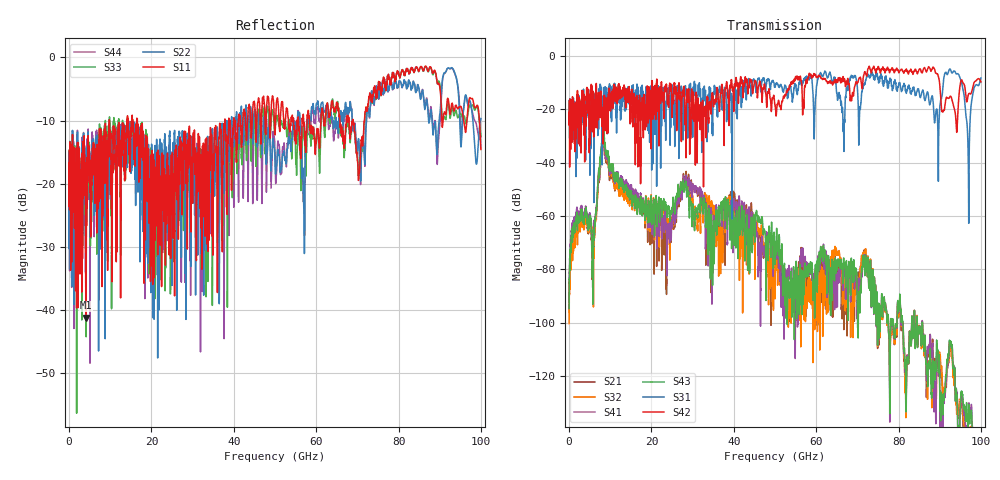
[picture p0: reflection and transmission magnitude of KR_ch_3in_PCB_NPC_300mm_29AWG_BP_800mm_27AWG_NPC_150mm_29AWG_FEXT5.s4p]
# GHz S RI R 45
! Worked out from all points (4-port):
!   4000 points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, 25 MHz to 100 GHz, reference 45 ohm
!   strongest paths, dB at 25 MHz, 25.02 GHz, 50.02 GHz, 75.03 GHz, 100 GHz:
!     S42: -21.2, -20.7, -18.6, -4.1, -9.8
!     S31: -21.3, -12.1, -11.5, -8.0, -8.3
!     S43: -94.7, -58.5, -72.8, -94.6, -158.5
!     S41: -92.2, -62.3, -71.0, -94.8, -150.9
!     S32: -100.3, -63.0, -83.5, -95.3, -162.7
!     S21: -96.2, -60.9, -74.2, -95.6, -162.4
!   lowest |S11| = -41.3 dB at 4.075 GHz (marker M1), VSWR 1.02, Z = 44.6 - j0.641 ohm
!   |S11| at or under -10 dB: start of sweep to 9.799 GHz; 9.805 GHz to 14.12 GHz (4.315 GHz wide, 36.1 % of centre); 16.58 GHz to 37.83 GHz (21.26 GHz wide, 78.1 % of centre)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
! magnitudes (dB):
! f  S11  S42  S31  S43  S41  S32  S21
! 25 MHz  -16.7  -21.2  -21.3  -94.7  -92.2  -100.3  -96.2
! 4.075 GHz  -41.3  -21.9  -35.0  -57.4  -56.6  -59.3  -59.0
! 8.375 GHz  -12.8  -19.1  -17.5  -28.2  -29.8  -29.5  -31.2
! 23.27 GHz  -24.1  -11.9  -24.6  -56.2  -59.1  -61.7  -61.0
! 28.6 GHz  -15.4  -13.1  -16.5  -52.7  -50.5  -50.4  -49.2
! 49.15 GHz  -7.3  -20.6  -10.1  -62.8  -67.8  -75.9  -80.7
! 100 GHz  -14.6  -9.8  -8.3  -158.5  -150.9  -162.7  -162.4
